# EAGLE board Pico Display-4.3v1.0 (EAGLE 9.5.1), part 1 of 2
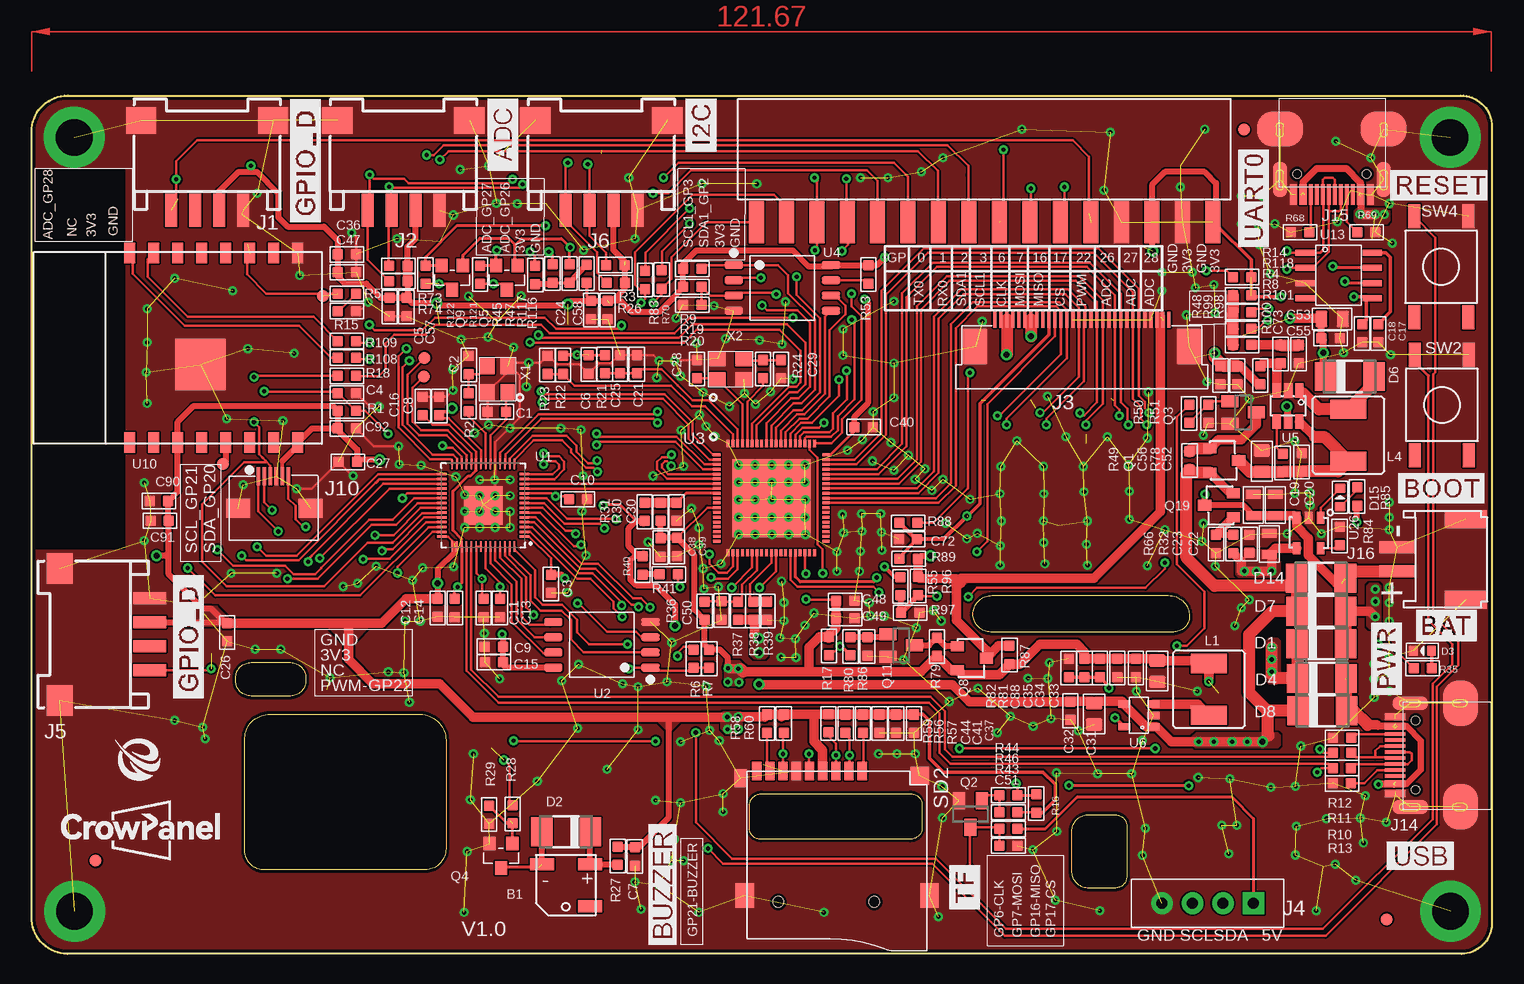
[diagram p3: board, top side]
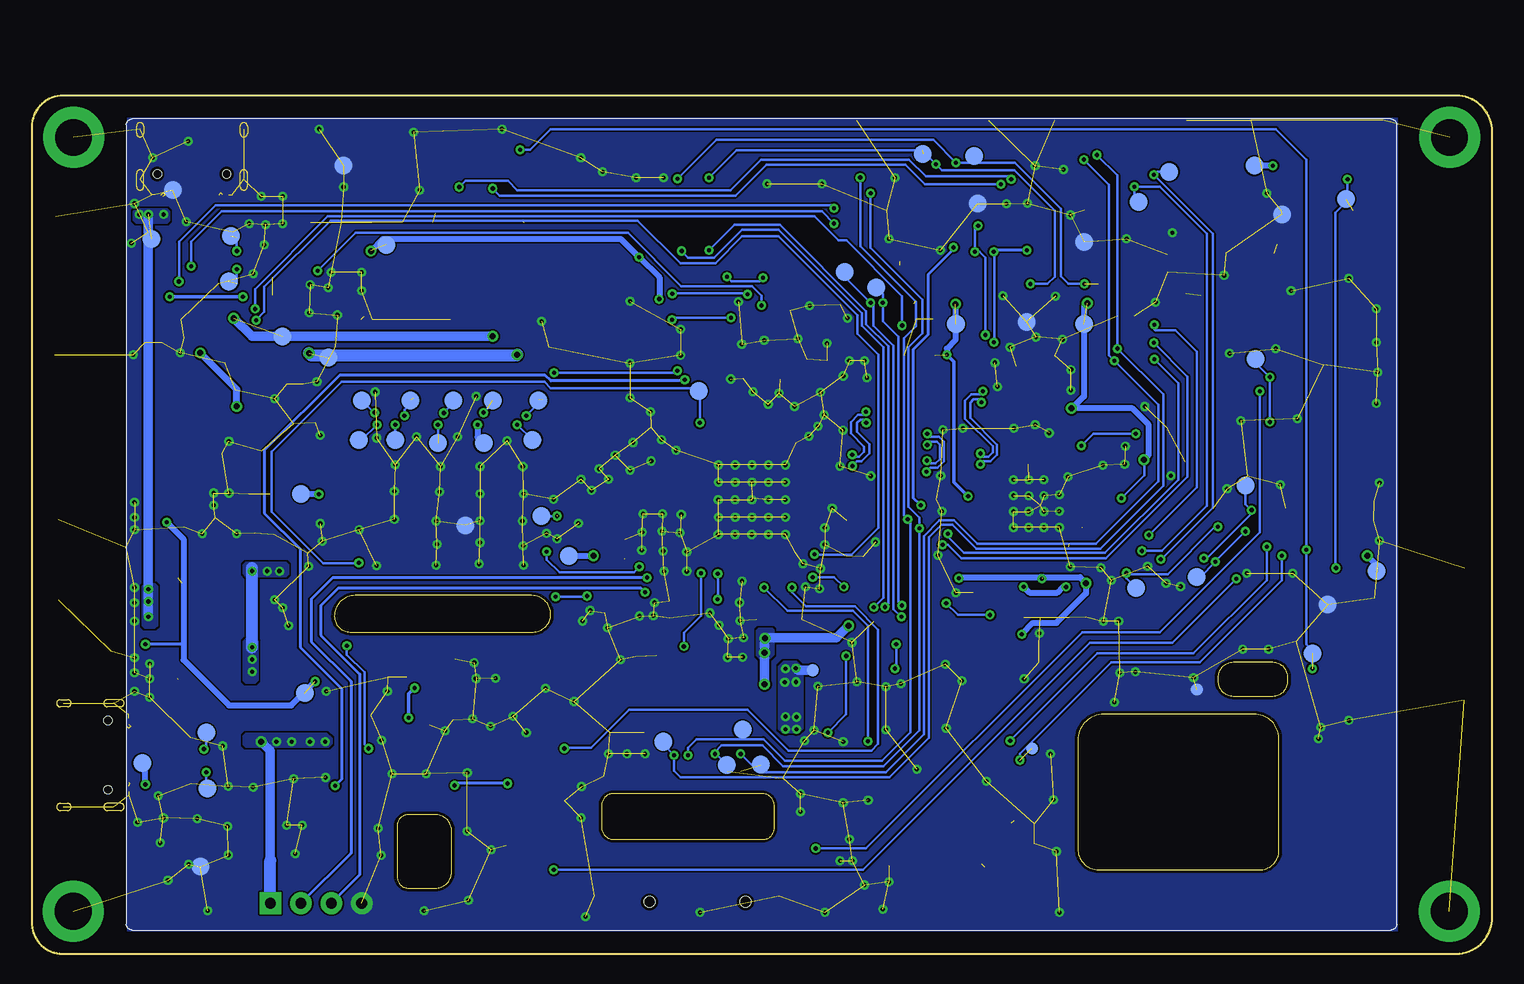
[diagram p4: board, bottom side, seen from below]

Size 121.74 x 71.53 mm. Coordinates in mm from the lower left corner, seen from the top.
Outline: 119.2,0 2.99,0 arc-90 0,3.07 0,68.5 arc-90 3.02,71.53 119.13,71.53 arc-90 121.74,68.94 121.74,2.64 arc-90 119.2,0
Outline: 73.25,9.55 60.77,9.55 arc-90 59.84,10.48 59.84,12.33 arc-90 60.88,13.36 73.25,13.36 arc-90 74.24,12.37 74.24,10.54 arc-90 73.25,9.55
Outline: 91.29,10.74 91.29,6.38 arc-90 90.32,5.49 88.14,5.49 arc-90 86.74,6.78 86.74,10.34 arc-90 88.14,11.58 90.32,11.58 arc-90 91.29,10.74
Outline: 95.21,26.82 79.96,26.82 arc-90 78.49,28.3 arc-90 80.06,29.87 94.79,29.87 arc-90 96.52,28.14 arc-90 95.21,26.82
Outline: 17.78,8.74 17.78,17.81 arc-90 19.68,19.96 32.39,19.96 arc-90 34.54,17.81 34.54,8.74 arc-90 32.81,7.01 19.26,7.01 arc-90 17.78,8.74
Outline: 21.59,21.49 18.29,21.49 arc-90 17.02,22.76 17.02,23.01 arc-90 18.29,24.28 21.59,24.28 arc-90 22.86,23.01 22.86,22.76 arc-90 21.59,21.49
Copper layers (1*16): Top 0.035mm / dielectric 1.5mm / Bottom 0.035mm
Design rules "default1 *": minimum track width 0.2mm, minimum drill 0.3mm, track to track 6mil, track to pad 4mil, pad to pad 4mil, via to via 6mil, smd to smd 6mil, copper to edge 10mil, drill to drill 4mil, minimum pad ring 10mil, minimum via ring 8mil, stop-mask expansion 4mil, vias tented up to drill 100mil, thermal gap 10mil
Net classes: 0 default: width 0.152 mm, drill 0.305 mm, clearance 0.152 mm; 1 PWR: width 0.254 mm; 2 GND: width 0.203 mm; 3 RS485: width 0.203 mm, clearance 0.203 mm; 4 USB: width 0.203 mm, clearance 0.152 mm; 5 ANT: width 0.889 mm, clearance 0.203 mm; 6 DVI-D0: width 0.203 mm, clearance 0.406 mm to class 0, clearance 0.203 mm
tRestrict: 10 lines

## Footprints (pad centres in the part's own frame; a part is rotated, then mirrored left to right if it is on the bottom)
BEEP_5025 = smd 2 x 1: 1 -2,-1.75; 2 2,-1.75; 3 -2,1.75
A_XBJ_0603 = smd 0.889 x 0.889: 1 -0.762,0; 2 0.762,0
0603 = smd 0.889 x 0.889: 1 -0.762,0; 2 0.762,0
0805_S = smd 0.762 x 1.27: 1 -0.889,0; 2 0.889,0
C0603 = smd 0.889 x 0.889: 1 -0.762,0; 2 0.762,0
A_XBJ_0805 = smd 1.016 x 1.397: 1 -0.889,0; 2 0.889,0
DISCRETE_C0603 = smd 0.889 x 0.889: 1 -0.762,0; 2 0.762,0
0805 = smd 1.016 x 1.397: 1 -0.889,0; 2 0.889,0
DO-214AC = smd 1.8 x 2.4: A 2.025,0; C -2.025,0
DISCRETE_D0603 = smd 0.762 x 0.889: + -0.762,0; - 0.762,0
CONNECTOR_4P-SMD-2.0-90D = smd 1.01 x 2.74: 1 -3,-0.1; 2 -1,-0.1; 3 1,-0.1; 4 3,-0.1 | smd 2.54 x 2.184: SS1 -5.5,7.4; SS2 5.5,7.4
FPC-30P-0.5 = smd 0.3 x 1.3: 1 9.75,2.54; 2 9.25,2.54; 3 8.75,2.54; 4 8.25,2.54; 5 7.75,2.54; 6 7.25,2.54; 7 6.75,2.54; 8 6.25,2.54; 9 5.75,2.54; 10 5.25,2.54; 11 4.75,2.54; 12 4.25,2.54; 13 3.75,2.54; 14 3.25,2.54; 15 2.75,2.54; 16 2.25,2.54; 17 1.75,2.54; 18 1.25,2.54; 19 0.75,2.54; 20 0.25,2.54; 21 -0.25,2.54; 22 -0.75,2.54; 23 -1.25,2.54; 24 -1.75,2.54; 25 -2.25,2.54; 26 -2.75,2.54; 27 -3.25,2.54; 28 -3.75,2.54; 29 -4.25,2.54; 30 -4.75,2.54 | smd 2 x 3: 31 -6.4,0.29; 32 11.4,0.29
CON_4PIN_DIP_P2.54 = drill 0.9 pad 1.8 square: P$1 -3.81,0 | drill 0.9 pad 1.8: P$2 -1.27,0; P$3 1.27,0; P$4 3.81,0
2.54-16P-WOTIE = smd 1.25 x 3.5: 1 -18.999,-5.572; 2 -16.51,-5.572; 3 -13.97,-5.572; 4 -11.43,-5.572; 5 -8.89,-5.572; 6 -6.35,-5.572; 7 -3.81,-5.572; 8 -1.27,-5.572; 9 1.27,-5.572; 10 3.81,-5.572; 11 6.35,-5.572; 12 8.89,-5.572; 13 11.43,-5.572; 14 13.97,-5.572; 15 16.51,-5.572; 16 19.05,-5.572
FPC-6PIN-0.5MM = smd 0.3 x 1.5: 1 -1.31,2.184; 2 -0.81,2.184; 3 -0.31,2.184; 4 0.19,2.184; 5 0.69,2.184; 6 1.19,2.184 | smd 2 x 1.6: 7 -3.01,-0.496; 8 3.036,-0.496
KEVIN_3.0TYPEC-SMD = smd 0.3 x 1.7: A1 -3.35,0.5; A4 -2.55,0.5; A5 -1.25,0.5; A6 -0.25,0.5; A7 0.25,0.5; A8 1.25,0.5; A9 2.55,0.5; A12 3.35,0.5; B1 3.05,0.5; B4 2.25,0.5; B5 1.75,0.5; B6 0.75,0.5; B7 -0.75,0.5; B8 -1.75,0.5; B9 -2.25,0.5; B12 -3.05,0.5 | smd 1.143 x 2.921: P$6 -4.318,-0.762; P$7 4.318,-0.762 | smd 3.81 x 2.921: P$8 -4.318,-4.953; P$9 4.318,-4.953 | hole 0.68: -2.89,-1.22; 2.89,-1.22
PH2.0WT-2PIN = smd 1 x 3: P$1 -1,0; P$2 1,0 | smd 1.5 x 3.5: P$3 -3.35,-5.7; P$4 3.35,-5.7
CD54_CD54 = smd 3 x 1.6: 1 0,2.159; 2 0,-2.159
PAD-1.0MM = smd 1 x 1: P$1 0,0
CROWPI_POW_PAD-1.0MM = smd 1 x 1: P$1 0,0
PAD-1.5MM = smd 1.5 x 1.5: P$1 0,0
SOT-23 = smd 1.1 x 0.8: 1 1.2,-1; 2 1.2,1 | smd 1.1 x 0.9: 3 -1.2,0
SPARKFUN_SOT23 = smd 1 x 1.4: 1 -0.95,-1.1; 2 0.95,-1.1; 3 0,1.1
DISCRETE_SOT23$1 = smd 1.016 x 1.143: 1 -0.95,-1.016; 2 0.95,-1.016; 3 0,1.016
SOT23 = smd 1.016 x 1.143: 1 -0.889,-1.016; 2 0.889,-1.016; 3 0,1.016
DISCRETE_R0603 = smd 0.889 x 0.889: 1 -0.762,0; 2 0.762,0
R0603 = smd 0.889 x 0.889: 1 -0.762,0; 2 0.762,0
9P-SMD-W/-RING = smd 1.524 x 0.762: 1 0,4.4; 2 0,3.3; 3 0,2.2; 4 0,1.1; 5 0,0; 6 0,-1.1; 7 0,-2.2; 8 0,-3.3; 9 0,-4.4 | smd 1.524 x 1.016: G1 0.6,-5.746 | smd 2.032 x 1.524: G2 10.373,-5.4; G3 10.373,10 | smd 1.524 x 1.524: G4 0.392,9.181 | hole 0.889: 10.9,-2.6; 10.9,5.4
KEY-6 = smd 2 x 1: 1 -4.2,2.25; 2 -4.2,-2.25; 3 4.2,-2.25; 4 4.2,2.25
3M-5 = drill 3.048 pad 5.08: 1 0,0
RP2040_QFN-56 = smd 0.875 x 0.2: 1 -3.437,2.6; 2 -3.437,2.2; 3 -3.437,1.8; 4 -3.437,1.4; 5 -3.437,1; 6 -3.437,0.6; 7 -3.437,0.2; 8 -3.437,-0.2; 9 -3.437,-0.6; 10 -3.437,-1; 11 -3.437,-1.4; 12 -3.437,-1.8; 13 -3.437,-2.2; 14 -3.437,-2.6; 29 3.437,-2.6; 30 3.437,-2.2; 31 3.437,-1.8; 32 3.437,-1.4; 33 3.437,-1; 34 3.437,-0.6; 35 3.437,-0.2; 36 3.437,0.2; 37 3.437,0.6; 38 3.437,1; 39 3.437,1.4; 40 3.437,1.8; 41 3.437,2.2; 42 3.437,2.6 | smd 0.2 x 0.875: 15 -2.6,-3.437; 16 -2.2,-3.437; 17 -1.8,-3.437; 18 -1.4,-3.437; 19 -1,-3.437; 20 -0.6,-3.437; 21 -0.2,-3.437; 22 0.2,-3.437; 23 0.6,-3.437; 24 1,-3.437; 25 1.4,-3.437; 26 1.8,-3.437; 27 2.2,-3.437; 28 2.6,-3.437; 43 2.6,3.437; 44 2.2,3.437; 45 1.8,3.437; 46 1.4,3.437; 47 1,3.437; 48 0.6,3.437; 49 0.2,3.437; 50 -0.2,3.437; 51 -0.6,3.437; 52 -1,3.437; 53 -1.4,3.437; 54 -1.8,3.437; 55 -2.2,3.437; 56 -2.6,3.437 | smd 3.2 x 3.2: EPAD 0,0
SELF_SOIC-8-208MIL = smd 1.5 x 0.635: 1 -4.05,1.905; 2 -4.05,0.635; 3 -4.05,-0.635; 4 -4.05,-1.905; 5 4.05,-1.905; 6 4.05,-0.635; 7 4.05,0.635; 8 4.05,1.905
RTD2281CL-MQFN-76 = smd 0.6 x 0.25: P$1 -4.55,3.6; P$2 -4.55,3.2; P$3 -4.55,2.8; P$4 -4.55,2.4; P$5 -4.55,2; P$6 -4.55,1.6; P$7 -4.55,1.2; P$8 -4.55,0.8; P$9 -4.55,0.4; P$10 -4.55,0; P$11 -4.55,-0.4; P$12 -4.55,-0.8; P$13 -4.55,-1.2; P$14 -4.55,-1.6; P$15 -4.55,-2; P$16 -4.55,-2.4; P$17 -4.55,-2.8; P$18 -4.55,-3.2; P$19 -4.55,-3.6; P$39 4.55,-3.6; P$40 4.55,-3.2; P$41 4.55,-2.8; P$42 4.55,-2.4; P$43 4.55,-2; P$44 4.55,-1.6; P$45 4.55,-1.2; P$46 4.55,-0.8; P$47 4.55,-0.4; P$48 4.55,0; P$49 4.55,0.4; P$50 4.55,0.8; P$51 4.55,1.2; P$52 4.55,1.6; P$53 4.55,2; P$54 4.55,2.4; P$55 4.55,2.8; P$56 4.55,3.2; P$57 4.55,3.6 | smd 0.25 x 0.6: P$20 -3.6,-4.55; P$21 -3.2,-4.55; P$22 -2.8,-4.55; P$23 -2.4,-4.55; P$24 -2,-4.55; P$25 -1.6,-4.55; P$26 -1.2,-4.55; P$27 -0.8,-4.55; P$28 -0.4,-4.55; P$29 0,-4.55; P$30 0.4,-4.55; P$31 0.8,-4.55; P$32 1.2,-4.55; P$33 1.6,-4.55; P$34 2,-4.55; P$35 2.4,-4.55; P$36 2.8,-4.55; P$37 3.2,-4.55; P$38 3.6,-4.55; P$58 3.6,4.55; P$59 3.2,4.55; P$60 2.8,4.55; P$61 2.4,4.55; P$62 2,4.55; P$63 1.6,4.55; P$64 1.2,4.55; P$65 0.8,4.55; P$66 0.4,4.55; P$67 0,4.55; P$68 -0.4,4.55; P$69 -0.8,4.55; P$70 -1.2,4.55; P$71 -1.6,4.55; P$72 -2,4.55; P$73 -2.4,4.55; P$74 -2.8,4.55; P$75 -3.2,4.55; P$76 -3.6,4.55 | smd 6.5 x 6.5: P$77 0,0
SOT23-6 = smd 0.69 x 1.2: 1 -0.95,-1.3; 2 0,-1.3; 3 0.95,-1.3; 4 0.95,1.3; 5 0,1.3; 6 -0.95,1.3
CROWBOT_-V1.0-20220525_A_XBJ_SOT23-5 = smd 0.6 x 1: 1 -0.95,-1.2; 2 0,-1.2; 3 0.95,-1.2; 4 0.95,1.2; 5 -0.95,1.2
BW16 = smd 1.7 x 0.9: 1 0.1,16; 2 0.1,14; 3 0.1,12; 4 0.1,10; 5 0.1,8; 6 0.1,6; 7 0.1,4; 8 0.1,2; 9 15.9,2; 10 15.9,4; 11 15.9,6; 12 15.9,8; 13 15.9,10; 14 15.9,12; 15 15.9,14; 16 15.9,16 | smd 4.3 x 4.2: 17 6.6,10.1
SOP8 = smd 0.5 x 1.6: P$1 -1.905,-2.8; P$2 -0.635,-2.8; P$3 0.635,-2.8; P$4 1.905,-2.8; P$5 1.905,2.8; P$6 0.635,2.8; P$7 -0.635,2.8; P$8 -1.905,2.8
SOP23-5 = smd 1 x 0.635: 1 -1.27,1; 2 -1.27,0; 3 -1.27,-1; 4 1.27,-1; 5 1.27,1
A_XBJ_SMD3225 = smd 1.4 x 1.2: 1 -1.1,-0.85; 2 1.1,-0.85; 3 1.1,0.85; 4 -1.1,0.85

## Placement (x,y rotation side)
B1  BEEP_5025  [BEEP_5025]  44.55,5.73 180 top
C1  12PF  [A_XBJ_0603]  38.78,45.18 180 top
C2  12PF  [A_XBJ_0603]  36.45,49.08 270 top
C3  2.2UF  [A_XBJ_0603]  43.29,30.84 270 top
C4  4.7uF  [A_XBJ_0603]  26.3,46.72 0 top
C5  100NF  [A_XBJ_0603]  29.86,53.9 270 top
C6  2.2UF  [A_XBJ_0603]  46.45,49.12 270 top
C7  100NF  [A_XBJ_0603]  50.3,8.12 270 top
C8  100NF  [A_XBJ_0603]  33.99,45.67 90 top
C9  100NF  [A_XBJ_0603]  38.55,25.61 180 top
C10  100NF  [A_XBJ_0603]  45.55,37.89 0 top
C11  100NF  [A_XBJ_0603]  37.68,28.83 270 top
C12  100NF  [A_XBJ_0603]  33.85,28.84 270 top
C13  100NF  [A_XBJ_0603]  39.05,28.83 270 top
C14  100NF  [A_XBJ_0603]  35.28,28.82 270 top
C15  2.2UF  [A_XBJ_0603]  38.55,24.31 180 top
C16  2.2UF  [A_XBJ_0603]  32.62,45.67 90 top
C17  100nF  [0603]  112.27,51.71 90 top
C18  100nF  [0603]  110.91,51.71 90 top
C19  10uF  [0805_S]  101.86,37.41 270 top
C20  10uF  [0805_S]  103.68,37.41 270 top
C21  10UF  [A_XBJ_0603]  50.46,49.14 90 top
C22  10uF  [0805_S]  103.17,34.17 270 top
C23  100nF  [C0603]  101.53,34.17 90 top
C24  100nF  [0603]  46.63,53.67 90 top
C25  100NF  [A_XBJ_0603]  49.06,49.14 90 top
C26  100nF  [0603]  16.32,26.8 90 top
C27  100NF  [A_XBJ_0603]  26.36,41 180 top
C28  22PF  [A_XBJ_0603]  55.46,48.73 90 top
C29  22PF  [A_XBJ_0603]  62.46,48.73 90 top
C30  100NF  [A_XBJ_0603]  53.77,36.85 270 top
C31  22UF  [A_XBJ_0805]  88.58,20 90 top
C32  1UF  [A_XBJ_0603]  86.6,20.26 270 top
C33  22UF  [A_XBJ_0805]  93.84,23.56 90 top
C34  1UF  [A_XBJ_0603]  92.07,23.81 270 top
C35  100NF  [A_XBJ_0603]  90.51,23.81 270 top
C36  2.2UF  [A_XBJ_0603]  26.3,58.29 0 top
C37  4.7uF  [DISCRETE_C0603]  73.55,19.19 90 top
C38  10uF  [A_XBJ_0603]  52.44,33.87 270 top
C39  100NF  [A_XBJ_0603]  53.81,33.9 270 top
C40  10UF  [A_XBJ_0603]  69.37,43.9 0 top
C41  1uF  [DISCRETE_C0603]  72.08,19.19 90 top
C44  100nF  [C0603]  70.69,19.19 270 top
C47  100NF  [A_XBJ_0603]  26.3,56.81 0 top
C48  10UF  [A_XBJ_0603]  67.83,29.42 0 top
C49  100NF  [A_XBJ_0603]  67.83,27.99 0 top
C50  100NF  [A_XBJ_0603]  57.52,28.61 270 top
C51  100NF  [A_XBJ_0603]  81.43,9.01 0 top
C52  1uF  [0603]  105.87,40.98 270 top
C53  22uF  [0805]  108.42,52.91 180 top
C55  100nF  [0603]  108.29,51.3 180 top
C56  22uF  [0805]  102.56,41.05 270 top
C57  100nF  [0603]  31.25,53.91 90 top
C58  100nF  [0603]  48.02,53.66 90 top
C72  4.7uF/NC  [0603]  73.07,34.55 180 top
C73  1UF  [A_XBJ_0603]  105.62,49.98 270 top
C88  22PF  [A_XBJ_0603]  89.06,23.81 270 top
C90  100NF  [A_XBJ_0603]  10.63,37.74 0 top
C91  1UF  [A_XBJ_0603]  10.69,36.09 180 top
C92  100NF  [A_XBJ_0603]  26.3,43.79 0 top
D1  IN5817  [DO-214AC]  107.52,25.85 0 top
D2  ss14  [DO-214AC]  44.55,10.17 180 top
D3  [DISCRETE_D0603]  115.94,25.26 180 top
D4  IN5817  [DO-214AC]  107.57,22.95 0 top
D6  ss14  [DO-214AC]  109.89,48.12 0 top
D7  IN5817  [DO-214AC]  107.51,28.55 0 top
D8  IN5817  [DO-214AC]  107.6,20.26 0 top
D14  IN5817  [DO-214AC]  107.49,31.3 0 top
D15  [DISCRETE_D0603]  109.08,38.03 90 top
J1  [CONNECTOR_4P-SMD-2.0-90D]  14.64,62.05 0 top
J2  [CONNECTOR_4P-SMD-2.0-90D]  31.01,62.05 0 top
J3  [FPC-30P-0.5]  85.06,50.32 0 top
J4  [CON_4PIN_DIP_P2.54]  98.04,4.22 180 top
J5  [CONNECTOR_4P-SMD-2.0-90D]  9.75,26.62 90 top
J6  [CONNECTOR_4P-SMD-2.0-90D]  47.5,62.05 0 top
J7  2.54-16PIN-WOTIE  [2.54-16P-WOTIE]  79.43,66.52 0 top
J10  FPC-6PIN-0.5MM  [FPC-6PIN-0.5MM]  20.22,37.64 0 top
J14  USB_TYPE-C_16PIN3.0USB  [KEVIN_3.0TYPEC-SMD]  114.16,16.57 90 top
J15  USB_TYPE-C_16PIN3.0USB  [KEVIN_3.0TYPEC-SMD]  108.39,63.77 180 top
J16  PH2.0WT-2PIN  [PH2.0WT-2PIN]  113.85,32.87 90 top
L1  [CD54_CD54]  98.15,22.04 180 top
L4  [CD54_CD54]  109.78,43.22 180 top
P1  PADPAD-1.0MM  [PAD-1.0MM]  5.33,7.77 0 top
P11  CROWPI_POW_PADPAD-1.0MM  [CROWPI_POW_PAD-1.0MM]  32.7,48.1 90 top
P12  CROWPI_POW_PADPAD-1.0MM  [CROWPI_POW_PAD-1.0MM]  32.76,49.66 0 top
P13  CROWPI_POW_PADPAD-1.0MM  [CROWPI_POW_PAD-1.0MM]  56.65,23.64 90 bottom
P14  CROWPI_POW_PADPAD-1.0MM  [CROWPI_POW_PAD-1.0MM]  24.62,22.03 0 bottom
P38  CROWPI_POW_PADPAD-1.0MM  [CROWPI_POW_PAD-1.0MM]  38.36,17.12 0 bottom
P48  PADPAD-1.0MM  [PAD-1.0MM]  112.96,2.88 0 top
P49  PADPAD-1.0MM  [PAD-1.0MM]  101.06,68.7 0 top
P82  CROWPI_POW_PADPAD-1.0MM  [CROWPI_POW_PAD-1.0MM]  15.94,40.83 90 top
P83  CROWPI_POW_PADPAD-1.0MM  [CROWPI_POW_PAD-1.0MM]  24.31,54.84 90 top
PAD1  PAD  [PAD-1.5MM]  9.65,31.9 0 bottom
PAD2  PAD  [PAD-1.5MM]  69.09,17.68 90 bottom
PAD3  PAD  [PAD-1.5MM]  62.48,18.69 90 bottom
PAD4  PAD  [PAD-1.5MM]  63.8,15.75 90 bottom
PAD5  PAD  [PAD-1.5MM]  60.96,15.77 90 bottom
PAD6  PAD  [PAD-1.5MM]  38.82,52.67 180 bottom
PAD7  PAD  [PAD-1.5MM]  98.98,21.73 180 bottom
PAD8  PAD  [PAD-1.5MM]  29.49,62.66 0 bottom
PAD9  PAD  [PAD-1.5MM]  26.92,65.18 0 bottom
PAD10  PAD  [PAD-1.5MM]  42.9,62.53 180 bottom
PAD11  PAD  [PAD-1.5MM]  44.7,52.48 180 bottom
PAD12  PAD  [PAD-1.5MM]  47.47,66.68 90 bottom
PAD13  PAD  [PAD-1.5MM]  43.19,66.48 90 bottom
PAD14  PAD  [PAD-1.5MM]  34.04,59.33 180 bottom
PAD15  PAD  [PAD-1.5MM]  34.04,52.48 180 bottom
PAD16  PAD  [PAD-1.5MM]  20.57,39.01 0 bottom
PAD17  PAD  [PAD-1.5MM]  12.19,62.89 90 bottom
PAD18  PAD  [PAD-1.5MM]  17.53,61.62 180 bottom
PAD19  PAD  [PAD-1.5MM]  19.81,65.68 180 bottom
PAD20  PAD  [PAD-1.5MM]  14.99,25.04 90 bottom
PAD21  PAD  [PAD-1.5MM]  76.96,33.17 90 bottom
PAD22  PAD  [PAD-1.5MM]  85.6,35.71 90 bottom
PAD23  PAD  [PAD-1.5MM]  94.23,46.13 270 bottom
PAD24  PAD  [PAD-1.5MM]  94.49,42.82 270 bottom
PAD25  PAD  [PAD-1.5MM]  107.7,7.26 0 bottom
PAD26  PAD  [PAD-1.5MM]  91.44,42.82 90 bottom
PAD27  PAD  [PAD-1.5MM]  90.17,46.13 90 bottom
PAD28  PAD  [PAD-1.5MM]  112.52,15.9 0 bottom
PAD29  PAD  [PAD-1.5MM]  13.72,29.11 0 bottom
PAD30  PAD  [PAD-1.5MM]  87.88,42.57 90 bottom
PAD31  PAD  [PAD-1.5MM]  86.61,46.13 90 bottom
PAD32  PAD  [PAD-1.5MM]  95.76,65.68 90 bottom
PAD33  PAD  [PAD-1.5MM]  84.07,42.57 0 bottom
PAD34  PAD  [PAD-1.5MM]  83.31,46.13 0 bottom
PAD35  PAD  [PAD-1.5MM]  92.2,59.08 90 bottom
PAD36  PAD  [PAD-1.5MM]  80.01,42.82 0 bottom
PAD37  PAD  [PAD-1.5MM]  79.5,46.13 0 bottom
PAD38  PAD  [PAD-1.5MM]  66.14,46.92 90 bottom
PAD39  PAD  [PAD-1.5MM]  79.25,36.47 90 bottom
PAD40  PAD  [PAD-1.5MM]  100.84,51.46 0 bottom
PAD41  PAD  [PAD-1.5MM]  97.03,49.68 0 bottom
PAD42  PAD  [PAD-1.5MM]  29.69,30.51 90 bottom
PAD43  PAD  [PAD-1.5MM]  51.36,55.51 90 bottom
PAD44  PAD  [PAD-1.5MM]  53.99,56.82 90 bottom
PAD45  PAD  [PAD-1.5MM]  107.19,18.44 0 bottom
PAD46  PAD  [PAD-1.5MM]  107.11,13.79 90 bottom
PAD47  PAD  [PAD-1.5MM]  109.98,63.65 0 bottom
PAD48  PAD  [PAD-1.5MM]  111.76,59.59 0 bottom
PAD49  PAD  [PAD-1.5MM]  105.16,59.84 0 bottom
PAD50  PAD  [PAD-1.5MM]  105.31,56.03 0 bottom
PAD51  PAD  [PAD-1.5MM]  19.73,49.59 0 bottom
PAD52  PAD  [PAD-1.5MM]  24.64,31.39 0 bottom
PAD53  PAD  [PAD-1.5MM]  99.3,38.33 0 bottom
Q1  PMOS-3401-4A  [SOT-23]  99.42,41.11 180 top
Q2  S8050  [SPARKFUN_SOT23]  78.27,11.66 180 top
Q3  S8050  [SPARKFUN_SOT23]  101,45.12 270 top
Q4  S8050  [DISCRETE_SOT23$1]  39.13,8.18 180 top
Q5  2N7002  [SOT23]  39.62,56.35 180 top
Q8  PMOS-3401-4A  [SOT-23]  78.39,24.64 180 top
Q9  2N7002  [SOT23]  35.07,56.35 180 top
Q11  S8050  [SPARKFUN_SOT23]  72.5,25.71 270 top
Q19  PMOS-3401-4A  [SOT-23]  98.99,37.39 0 top
R1  10K  [DISCRETE_R0603]  26.3,45.26 180 top
R2  1K  [DISCRETE_R0603]  36.44,45.98 270 top
R3  1K  [DISCRETE_R0603]  48.67,57.4 0 top
R4  0R  [DISCRETE_R0603]  100.91,53.49 0 top
R5  OR/NC  [DISCRETE_R0603]  26.3,55.02 180 top
R6  1K  [DISCRETE_R0603]  55.18,24.6 90 top
R7  10K  [DISCRETE_R0603]  56.49,24.6 90 top
R8  0R/NC  [DISCRETE_R0603]  100.91,52.09 0 top
R9  10K  [DISCRETE_R0603]  55.07,57.07 180 top
R10  0R  [DISCRETE_R0603]  109.23,15.48 180 top
R11  0R  [DISCRETE_R0603]  109.25,16.76 180 top
R12  5.1K  [DISCRETE_R0603]  109.25,18.01 180 top
R13  5.1K  [DISCRETE_R0603]  109.23,14.21 0 top
R14  10K  [DISCRETE_R0603]  100.91,56.4 0 top
R15  1k  [DISCRETE_R0603]  26.3,53.57 180 top
R16  4.7K  [DISCRETE_R0603]  83.75,12.52 270 top
R17  4.7K  [DISCRETE_R0603]  66.48,25.65 90 top
R18  OR  [DISCRETE_R0603]  26.3,48.16 0 top
R19  1k  [DISCRETE_R0603]  55.07,55.6 180 top
R20  1K  [DISCRETE_R0603]  55.07,54.1 0 top
R21  OR  [DISCRETE_R0603]  47.79,49.14 90 top
R22  OR/L/NC  [DISCRETE_R0603]  44.3,49.09 90 top
R23  12K  [DISCRETE_R0603]  43,49.09 90 top
R24  0R  [DISCRETE_R0603]  60.96,48.73 270 top
R26  1K  [DISCRETE_R0603]  48.7,55.94 0 top
R27  100R  [DISCRETE_R0603]  48.87,8.17 90 top
R28  1K  [DISCRETE_R0603]  40.11,11.64 90 top
R29  10K  [DISCRETE_R0603]  38.15,11.6 90 top
R30  OR/NC  [DISCRETE_R0603]  52.44,36.84 270 top
R31  OR  [DISCRETE_R0603]  51.1,36.85 270 top
R32  1K  [DISCRETE_R0603]  100.19,34.15 270 top
R35  4.7K  [DISCRETE_R0603]  115.97,23.79 180 top
R36  OR/NC  [DISCRETE_R0603]  56.12,28.59 270 top
R37  OR/L  [DISCRETE_R0603]  58.89,28.59 270 top
R38  100k  [DISCRETE_R0603]  60.16,28.59 270 top
R39  200k  [DISCRETE_R0603]  61.33,28.59 90 top
R40  100k  [DISCRETE_R0603]  50.93,32.37 90 top
R41  1K  [DISCRETE_R0603]  53.13,31.62 180 top
R43  10K  [DISCRETE_R0603]  81.43,10.41 0 top
R44  10K  [R0603]  81.43,13.21 0 top
R45  4.7K  [DISCRETE_R0603]  41.99,56.59 270 top
R46  10K  [DISCRETE_R0603]  81.43,11.81 0 top
R47  4.7K  [DISCRETE_R0603]  43.41,56.69 270 top
R48  10R 1%  [DISCRETE_R0603]  99.12,48.21 270 top
R49  100K  [R0603]  96.53,41.11 90 top
R50  100R  [R0603]  96.5,45.02 90 top
R51  10k  [R0603]  98.1,45.02 90 top
R53  1K  [DISCRETE_R0603]  69.76,56.62 270 top
R55  0R  [DISCRETE_R0603]  72.44,30.63 270 top
R56  10K  [DISCRETE_R0603]  67.86,19.19 270 top
R57  10K  [DISCRETE_R0603]  69.3,19.19 270 top
R58  10K  [DISCRETE_R0603]  61.31,19.19 270 top
R59  10K  [DISCRETE_R0603]  66.44,19.21 270 top
R60  10K  [DISCRETE_R0603]  62.7,19.19 270 top
R66  10K  [DISCRETE_R0603]  98.74,34.15 90 top
R68  5.1K  [DISCRETE_R0603]  105.75,60.13 180 top
R69  5.1K  [DISCRETE_R0603]  111.27,60.13 180 top
R70  0R  [DISCRETE_R0603]  52.53,56.19 90 top
R73  1K  [DISCRETE_R0603]  30.59,56.05 0 top
R74  1K  [DISCRETE_R0603]  30.59,57.34 0 top
R78  4.7K  [DISCRETE_R0603]  104.3,40.92 270 top
R79  100K  [R0603]  75.48,25.6 90 top
R80  100K  [R0603]  68.28,25.63 270 top
R81  45.3K 1%  [DISCRETE_R0603]  87.78,23.81 270 top
R82  10K 1%  [DISCRETE_R0603]  86.45,23.81 270 top
R83  0R  [DISCRETE_R0603]  51.13,56.17 90 top
R84  2K  [DISCRETE_R0603]  109.04,34.82 90 top
R85  4.7K  [DISCRETE_R0603]  110.5,38.12 270 top
R86  100k  [R0603]  69.68,25.61 90 top
R87  0R/NC  [DISCRETE_R0603]  81.53,24.9 90 top
R88  0R  [DISCRETE_R0603]  73.09,35.93 0 top
R89  NC/1K  [DISCRETE_R0603]  73.11,32.93 0 top
R96  10K  [DISCRETE_R0603]  73.91,30.65 90 top
R97  10K/NC  [DISCRETE_R0603]  73.24,28.43 180 top
R98  2K 1%  [DISCRETE_R0603]  102.43,48.22 90 top
R99  10R 1%  [DISCRETE_R0603]  100.52,48.21 90 top
R100  24K 1%  [DISCRETE_R0603]  104.12,49.98 90 top
R101  4.7K 1%  [DISCRETE_R0603]  100.91,50.75 180 top
R108  OR  [DISCRETE_R0603]  26.3,49.69 180 top
R109  OR  [DISCRETE_R0603]  26.3,51.07 180 top
R116  OR/NC  [DISCRETE_R0603]  46.28,56.68 270 top
R117  0R  [DISCRETE_R0603]  44.85,56.69 90 top
R118  4.7K  [DISCRETE_R0603]  100.91,54.87 0 top
R121  OR/NC  [DISCRETE_R0603]  37.38,56.6 90 top
R122  OR/NC  [DISCRETE_R0603]  32.83,56.6 90 top
SD2  [9P-SMD-W/-RING]  64.85,15.23 270 top
SW2  KEY-6  [KEY-6]  117.58,45.75 270 top
SW4  KEY-6  [KEY-6]  117.5,57.25 270 top
T1  3M-5  [3M-5]  3.58,3.56 0 top
T2  3M-5  [3M-5]  3.56,68.05 0 top
T3  3M-5  [3M-5]  118.29,3.56 0 top
T4  3M-5  [3M-5]  118.26,68.05 0 top
U1  RP2040_RP2040  [RP2040_QFN-56]  37.66,37.37 180 top
U2  SELF_W25Q128JV  [SELF_SOIC-8-208MIL]  47.54,25.76 180 top
U3  [RTD2281CL-MQFN-76]  61.66,37.98 0 top
U4  SELF_W25Q128JV  [SELF_SOIC-8-208MIL]  62.58,55.5 0 top
U5  MT9201  [SOT23-6]  104.74,45.66 180 top
U6  RY3420  [CROWBOT_-V1.0-20220525_A_XBJ_SOT23-5]  92.31,19.87 90 top
U10  BW16  [BW16]  24.19,42.51 90 top
U13  CH340NSOP-8  [SOP8]  108.97,56.54 270 top
U26  4054A  [SOP23-5]  106.46,35.08 270 top
U$13  [LOGE-2.0]  2.77,8.28 0 top
U$26  [LOGLE]  5.97,13.32 0 top
X1  12MHZ_SMD3225  [A_XBJ_SMD3225]  38.84,47.89 90 top
X2  14.318MHZ_SMD3225  [A_XBJ_SMD3225]  58.26,48.73 0 top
